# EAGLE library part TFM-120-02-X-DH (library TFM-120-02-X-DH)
0.050" DOUBLE HORIZONTAL TERMINAL STRIP.
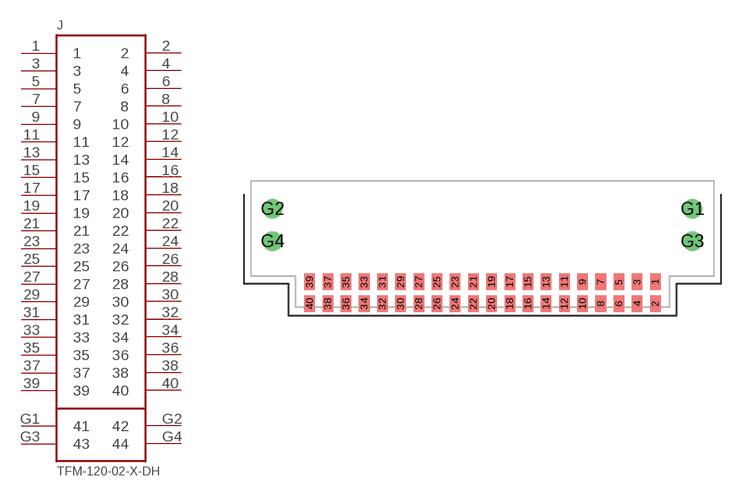
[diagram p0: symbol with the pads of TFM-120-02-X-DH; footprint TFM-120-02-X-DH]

Designator prefix J

## TFM-120-02-X-DH (Description: Connector, Header, 40 Position, 2row, 1.27mm; Digi-Key_Part_Number: SAM10153-ND; Digi-Key_Purchase_URL: https://www.digikey.com/product-detail/en/samtec-inc/TFM-120-02-L-DH/SAM10153-ND/6678890?utm_source=snapeda&utm_medium=aggregator&utm_campaign=symbol; MF: Samtec; MP: TFM-120-02-L-DH; Package: None)  [TFM-120-02-X-DH]
1  1
2  2
3  3
4  4
5  5
6  6
7  7
8  8
9  9
10  10
11  11
12  12
13  13
14  14
15  15
16  16
17  17
18  18
19  19
20  20
21  21
22  22
23  23
24  24
25  25
26  26
27  27
28  28
29  29
30  30
31  31
32  32
33  33
34  34
35  35
36  36
37  37
38  38
39  39
40  40
G1  41
G2  42
G3  43
G4  44

## Footprint TFM-120-02-X-DH (pad centres in mm)
0.050" DOUBLE HORIZONTAL TERMINAL STRIP.
smd 0.737 x 1.143: 1 12.065,-6.579; 2 12.065,-8.103; 3 10.795,-6.579; 4 10.795,-8.103; 5 9.525,-6.579; 6 9.525,-8.103; 7 8.255,-6.579; 8 8.255,-8.103; 9 6.985,-6.579; 10 6.985,-8.103; 11 5.715,-6.579; 12 5.715,-8.103; 13 4.445,-6.579; 14 4.445,-8.103; 15 3.175,-6.579; 16 3.175,-8.103; 17 1.905,-6.579; 18 1.905,-8.103; 19 0.635,-6.579; 20 0.635,-8.103; 21 -0.635,-6.579; 22 -0.635,-8.103; 23 -1.905,-6.579; 24 -1.905,-8.103; 25 -3.175,-6.579; 26 -3.175,-8.103; 27 -4.445,-6.579; 28 -4.445,-8.103; 29 -5.715,-6.579; 30 -5.715,-8.103; 31 -6.985,-6.579; 32 -6.985,-8.103; 33 -8.255,-6.579; 34 -8.255,-8.103; 35 -9.525,-6.579; 36 -9.525,-8.103; 37 -10.795,-6.579; 38 -10.795,-8.103; 39 -12.065,-6.579; 40 -12.065,-8.103
drill 0.838 pad 1.27: G1 14.656,-1.473; G2 -14.656,-1.473; G3 14.656,-3.734; G4 -14.656,-3.734

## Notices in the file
This work is licensed under a Creative Commons Attribution-ShareAlike 4.0 International License (CC BY-SA) with Design Exception 1.0
